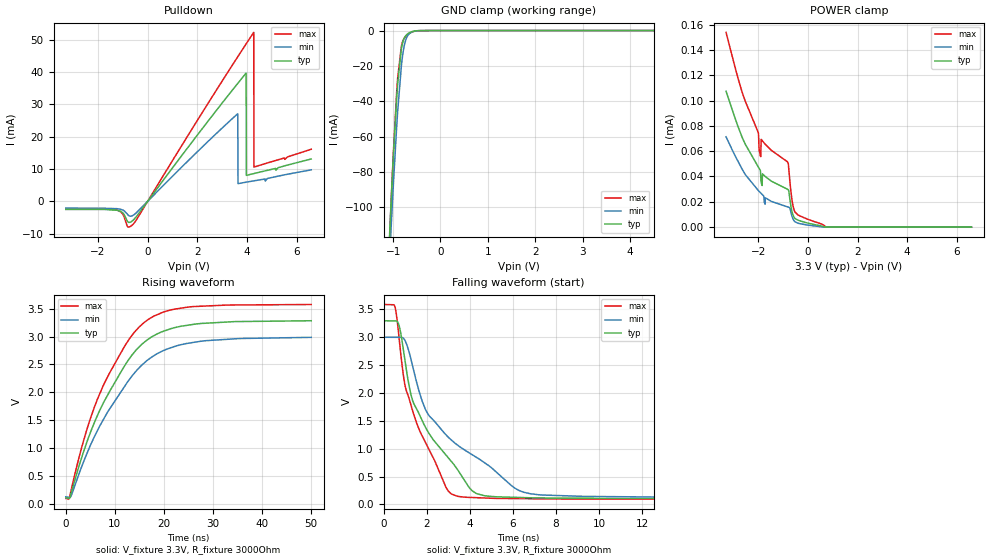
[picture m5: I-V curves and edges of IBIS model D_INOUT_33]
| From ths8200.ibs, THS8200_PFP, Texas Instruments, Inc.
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[Model]   D_INOUT_33
Model_type   I/O_open_drain
Polarity   Non-Inverting
Enable   Active-Low
Vinl = 1.15
Vinh = 2.3
Vmeas = 1.65
Vref = 0
Cref = 0pF
Rref = 3000
|   typ   min   max
|   (nom PVT)   (Fast PVT)   (slow PVT)
C_comp   1.174p   0.950p   1.418p
|C_comp (Hi state)   1.275p   1.071p   1.478p
|C_comp (Low state)   1.174p   0.950p   1.418p
| Where   nom PVT is  Nominal Process, 3.3V, 27C
|   Fast PVT is Strong Process, 3.6V, 0C
|   Slow PVT is Weak Process, 3.0V, 85C
[Voltage Range]   3.3   3   3.6
[Temperature Range]   27   85   0
[Pullup Reference]   3.3   3   3.6
[Pulldown Reference]   -0   -0   -0
[Power Clamp Reference]   3.3   3   3.6
[GND Clamp Reference]   -0   -0   -0
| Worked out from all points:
|   slope of the pulldown table from 0 to 0.495 V, typ, clamps not added: 96.3 ohm
|   GND clamp passes 1 mA (typ) near -0.64 V on its own axis
|   falling waveform, V_fixture 3.3V, R_fixture 3000Ohm: 20-80 % time 2.25ns typ, 3.49ns min, 1.62ns max; typ from 3.29 V to 0.102 V
|   rising waveform, V_fixture 3.3V, R_fixture 3000Ohm: 20-80 % time 10.4ns typ, 11.3ns min, 9.79ns max; typ from 0.102 V to 3.28 V
[Pulldown]
|   Voltage   I(typ)   I(min)   I(max)
-3.3V     -2.526mA   -2.103mA   -2.328mA
-1.251V   -2.75mA    -2.277mA   -2.706mA
-805.2mV  -6.315mA   -4.104mA   -7.877mA
-617.1mV  -6.066mA   -4.458mA   -7.33mA
3.62V     36.44mA    27.08mA    44.66mA
3.63V     36.53mA    27.08mA    44.78mA
3.64V     36.63mA    5.474mA    44.9mA
3.967V    39.73mA    5.923mA    48.76mA
3.977V    8.03mA     5.937mA    48.88mA
4.274V    8.59mA     6.333mA    52.35mA
4.283V    8.608mA    6.346mA    10.6mA
6.59V     13.12mA    9.75mA     16.13mA
[GND Clamp]
|   Voltage   I(typ)   I(min)   I(max)
-3.3V     -1.662A    -1.569A    -1.815A
-1.142V   -155.4mA   -166.8mA   -161.9mA
-1.043V   -96.72mA   -111.9mA   -97.53mA
-993.3mV  -69.98mA   -86.34mA   -68.46mA
-924mV    -37.81mA   -54.04mA   -34.44mA
-904.2mV  -30.26mA   -45.84mA   -26.87mA
-825mV    -10.13mA   -19.76mA   -8.749mA
-785.4mV  -5.697mA   -11.57mA   -5.388mA
-716.1mV  -2.426mA   -4.151mA   -2.793mA
-636.9mV  -980.7uA   -1.343mA   -1.29mA
-270.6mV  -22.84uA   -19.89uA   -41.19uA
6.59V     0A         0A         0A
[POWER Clamp]
|   Voltage   I(typ)   I(min)   I(max)
-3.3V     107.3uA    71.34uA    153.8uA
-2.656V   71.17uA    46uA       106.8uA
-2.003V   47.6uA     29.03uA    74.8uA
-1.904V   41.13uA    27.03uA    55.65uA
-1.884V   35.37uA    26.64uA    69.33uA
-1.845V   32.87uA    25.85uA    68.39uA
-1.835V   42.09uA    25.66uA    68.14uA
-825mV    29.94uA    16.01uA    51.63uA
-607.2mV  9.937uA    6.714uA    17.41uA
-409.2mV  5.583uA    3.182uA    9.765uA
749.1mV   0A         0A         0A
6.59V     0A         0A         0A
[Ramp]
R_load = 3000
|   typ   min   max
dV/dt_r   1.90959/1.03984e-08   1.71847/1.12856e-08   2.09057/9.79333e-09
dV/dt_f   1.91331/2.25351e-09   1.72374/3.49199e-09   2.0939/1.61843e-09
[Falling Waveform]
V_fixture = 3.3V
V_fixture_min = 3V
V_fixture_max = 3.6V
R_fixture = 3000Ohm
C_fixture = 0F
|   Time   V(typ)   V(min)   V(max)
0s        3.291V     2.995V     3.582V
527ps     3.288V     2.994V     3.537V
714.8ps   3.207V     2.994V     2.99V
979.5ps   2.607V     2.945V     2.157V
1.53ns    1.711V     2.19V      1.459V
2.092ns   1.282V     1.599V     995mV
3.427ns   624.9mV    1.065V     146.8mV
4.303ns   195.8mV    845.1mV    121.8mV
7.363ns   116.8mV    169.3mV    101mV
50ns      101.7mV    122.2mV    91.96mV
[Rising Waveform]
V_fixture = 3.3V
V_fixture_min = 3V
V_fixture_max = 3.6V
R_fixture = 3000Ohm
C_fixture = 0F
|   Time   V(typ)   V(min)   V(max)
0s        101.8mV    121.9mV    91.81mV
700.6ps   92.81mV    112.1mV    93.35mV
1.13ns    199.8mV    144.9mV    257mV
4.087ns   1.051V     852.8mV    1.271V
7.439ns   1.769V     1.475V     2.081V
11.92ns   2.466V     2.098V     2.818V
15.92ns   2.893V     2.522V     3.251V
20.54ns   3.115V     2.773V     3.458V
27.54ns   3.235V     2.916V     3.545V
50ns      3.284V     2.986V     3.576V
